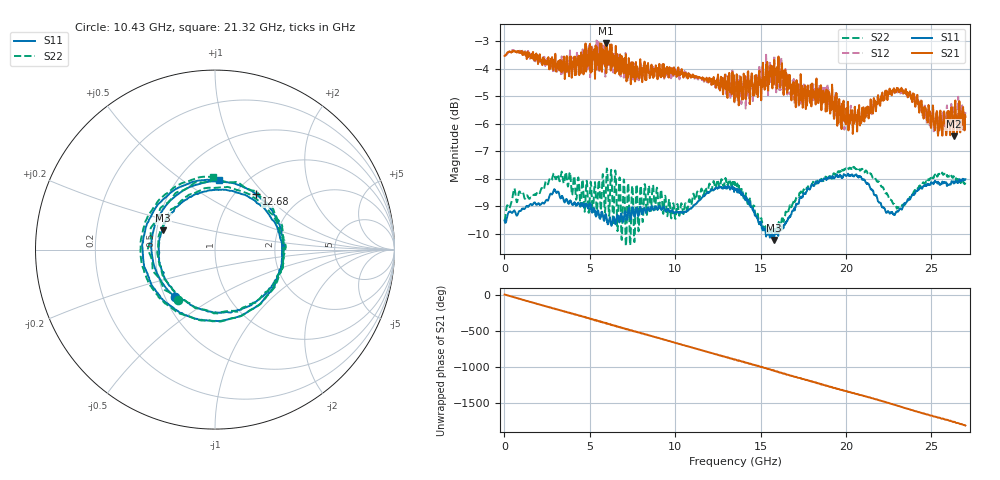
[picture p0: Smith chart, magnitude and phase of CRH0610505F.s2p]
!Agilent Technologies,N5224A,MY51441447,A.10.00.00
!Agilent N5224A: A.10.00.00
!Date: Thursday, November 05, 2015 12:16:56
!Correction: S11(Full 2 Port(1,2))
!S21(Full 2 Port(1,2))
!S12(Full 2 Port(1,2))
!S22(Full 2 Port(1,2))
!S2P File: Measurements: S11, S21, S12, S22:
# Hz S  RI  R 50
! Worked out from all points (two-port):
!   1601 points, 10 MHz to 27 GHz, reference 50 ohm
!   highest |S21| = -3.08 dB at 5.931 GHz (marker M1); lowest = -6.5 dB at 26.31 GHz (marker M2)
!   |S21| within 3 dB of the highest: start of sweep to 19.74 GHz; 20.67 GHz to 24.97 GHz (4.296 GHz wide, 18.8 % of centre)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
!   lowest |S11| = -10.2 dB at 15.8 GHz (marker M3), VSWR 1.89, Z = 27.1 + j6.46 ohm
!   |S11| at or under -10 dB: 15.30656 GHz to 15.3358 GHz (29.24 MHz wide, 0.191 % of centre); 15.47 GHz to 15.87 GHz (400.7 MHz wide, 2.56 % of centre); 15.96589 GHz to 15.98974 GHz (23.84 MHz wide, 0.149 % of centre)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
!   |S22| runs from -10.5 to -7.6 dB; largest |S21 - S12| = 0.081
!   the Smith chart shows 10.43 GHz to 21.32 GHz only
!   S11 on the Smith chart (normalised r, x): 10.43 GHz: 0.56, -0.34; 12.68 GHz: 1.23, +0.89; 21.32 GHz: 0.77, +0.70
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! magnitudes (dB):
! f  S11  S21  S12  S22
! 10 MHz  -9.5  -3.5  -3.6  -9.5
! 532.9 MHz  -9.2  -3.4  -3.3  -8.4
! 1.545 GHz  -8.9  -3.6  -3.5  -8.7
! 2.979 GHz  -8.4  -3.5  -3.8  -8.0
! 4.514 GHz  -8.9  -3.7  -3.5  -8.5
! 5.931 GHz  -9.3  -3.1  -3.6  -8.7
! 7.247 GHz  -9.2  -4.2  -4.0  -8.2
! 9.018 GHz  -9.1  -4.1  -4.3  -9.0
! 10.43 GHz  -9.2  -4.1  -4.2  -9.1
! 12.68 GHz  -8.3  -4.3  -4.5  -8.1
! 13.51 GHz  -8.4  -4.7  -4.6  -8.2
! 15.8 GHz  -10.2  -3.7  -3.7  -10.0
! 17.11 GHz  -8.9  -4.4  -4.4  -8.7
! 18.01 GHz  -8.2  -4.7  -4.8  -8.2
! 18.8 GHz  -8.0  -5.2  -4.9  -7.9
! 20.05 GHz  -7.9  -5.6  -5.6  -7.6
! 21.32 GHz  -8.2  -5.7  -5.6  -7.9
! 22.51 GHz  -9.2  -4.9  -4.8  -8.7
! 23.17 GHz  -9.1  -4.8  -4.9  -9.1
! 25.28 GHz  -8.1  -5.8  -5.7  -7.9
! 26.31 GHz  -8.1  -6.5  -5.8  -7.9
! 27 GHz  -8.0  -5.8  -5.7  -8.1
